ORGANIZATION_BLOCK MAIN:OB1
TITLE=Miscelatore a 4 ingressi
//Simulatore: 13
//Versione: 1.0
//Data:08/01/2002
//--------------- Descrizione dell'impianto -----------------------
//Un impianto di miscelazione automatico deve dosare opportunamente
//e mescolare 4 liquidi diversi. I singoli liquidi vengono prelevati
//da 4 serbatoi separati tramite il comando di 4 elettrovalvole
//(YV1..YV4).
//La pompa P1 pompa i liquidi in un serbatoio S dove il motore M2
//effettua l'operazione di mescolazione.
//Gli interruttori di di prossimità SL1..SL4, impostabili come
//posizione danno il livello di riempimento del serbatoio S,
//l'interruttore di prossimità SL0 segnala quando il serbatoio è vuoto.
//
//--------- Funzionamento dell'impianto ---------------------------
//Il processo di miscelazione inizia quando l'operatore preme il
//pulsante di start SB1. Per poter avviare il ciclo di riempimento
//occore che il sebatoio sia vuoto, l'elettrovalvola YV5 di scarico
//sia chiusa (non eccitata) e non siano intervenute le protezioni
//temiche dei motori M1 e M2.
//Se sono verificate queste condizioni la lampada di start HL2 si
//accende la pompa  P1 e il mescolatore M2 vengono inseriti.
//L'elettrovalvola YV1 si apre ed il liquido A viene immesso nel
//serbatoio S fino a quando il livello raggiunge l'interruttore di
//prossimità SL1.
//L'elettrovalvola YV1 si chiude e l'elettrovalvola YV2 (prodotto B)
//si apre fino a quando il livello raggiunge l'interruttore di
//prossimità SL2.Analogo procedimento si ha per i liquidi C e D.
//
//Quando si chiude l'elettrovalvola YV4, la pompa P1 viene disinserita.
//Dieci secondi dopo la chiusura dell'elettrovalvola YV4, si spegne la
//lampada di start HL2 e la lampada di fine ciclo HL6 si accende per
//segnalare agli operatori la fine del processo di miscelazione.
//
//Dopo l'accensione della lampada HL6, l'operatore può premere il
//pulsante di stop SB2. Il mescolatore M2 viene disinserito e la
//lampada HL6 si spegne, il serbatoio può essere svuotato.
//Se la lampada HL6 non si accende, il pulsante di stop non è abilitato.
//
//A questo punto può quindi iniziare la fase di scarico comandata dal
//selettore SB4 che azionerà l'elettrovalvola YV5; a scarico completato
//l'interruttore di prossimità SL0 segnalerà la condizione di
//serbatoio vuoto.
//
//L'impianto viene fermato se viene premuto il pulsante di emergenza
//SB5 o scatta uno dei due interuttori termici di sovracorrente
//FR1 o FR2; l'intervento dei termici viene segnalato da due lampade
//HL7 e Hl8. Le lampade HL3, HL4 e HL5 segnalano rispettivamente:
//HL3 Pompa Carico ON;
//HL4 Mecolatore M1 ON
//HL5 Elettrovalvola di scarico YV5 eccitata.

BEGIN
NETWORK 1 //Attivazione merker si STOP
//
//COMMENTI DEL SEGMENTO
//
LD I1.3
A I1.0
A I1.1
= M0.1

NETWORK 2 //Set marker Fase 1
//
LD I0.0
AN M0.0
AN I0.6
AN I1.2
S M1.1 1

NETWORK 3 //Reset Merker fase 1
//
LD M1.2
ON M0.1
R M1.1 1

NETWORK 4 //Set Merker fase 2
//
LD M1.1
AN I0.1
S M1.2 1

NETWORK 5 //Reset Merker fase 2
//
LD M1.3
ON M0.1
R M1.2 1

NETWORK 6 //Set Merker fase 3
//
LD M1.2
AN I0.2
S M1.3 1

NETWORK 7 //Reset Merker Fase 3
//
LD M1.4
ON M0.1
R M1.3 1

NETWORK 8 //Set Merker fase 4
//
LD M1.3
AN I0.3
S M1.4 1

NETWORK 9 //Reset Merker Fase 4
//
LD M1.5
ON M0.1
R M1.4 1

NETWORK 10 //Set Merker fase 5
//
LD M1.4
AN I0.4
S M1.5 1

NETWORK 11 //Reset Merker fase 5
//
LD M1.6
ON M0.1
R M1.5 1

NETWORK 12 //Gestione merker fase 6
//
LDN I0.5
A T37
A M1.5
A M0.1
= M1.6

NETWORK 13 //Set Merker Start
//
LD M1.1
S M0.0 1

NETWORK 14 //Reset Merker Start
//
LD M1.6
ON M0.1
R M0.0 1

NETWORK 15 //Set Lampada ciclo
//
LD M1.1
S Q1.1 1

NETWORK 16 //Reset Lampada ciclo
//
LD T37
ON M0.1
R Q1.1 1

NETWORK 17 //Comando Set Miscelatore
//
LD M1.1
S Q0.4 1

NETWORK 18 //Comando Reset Miscelatore
//
LD M1.6
ON M0.1
R Q0.4 1

NETWORK 19 //Comando Set Pompa Carico
//
LD M1.1
S Q0.5 1

NETWORK 20 //Comando Reset Pompa Carico
//
LD M1.5
ON M0.1
R Q0.5 1

NETWORK 21 //Carico Prodotto A
//
LD M1.1
A I0.1
= Q0.0

NETWORK 22 //Carico Prodotto B
//
LD M1.2
A I0.2
= Q0.1

NETWORK 23 //Carico Prodotto C
//
LD M1.3
A I0.3
= Q0.2

NETWORK 24 //Carico Prodotto D
//
LD M1.4
A I0.4
= Q0.3

NETWORK 25 //Temporizzazione Fine ciclo
//
LD M1.5
TON T37 +50

NETWORK 26 //Lampada fine ciclo
//
LD T37
= Q1.2

NETWORK 27 //Scarico Miscela manuale e segnalazione
//
LD I1.2
AN Q1.1
AN Q1.2
= Q0.6
= Q1.3

NETWORK 28 //Segnalazione Termico Motore Pompa
//
LDN I1.0
= Q1.6

NETWORK 29 //Segnalazione termico mescolatore
//
LDN I1.1
= Q1.7

NETWORK 30 //Segnalazione Pompa ON
//
LD Q0.5
= Q1.4

NETWORK 31 //Segnalazione Mescolatore ON
//
LD Q0.4
= Q1.5

END_ORGANIZATION_BLOCK

